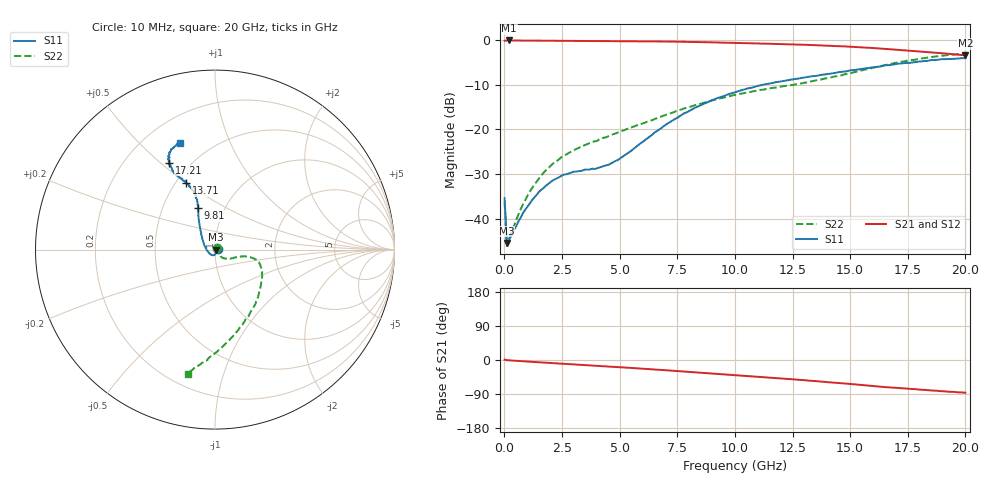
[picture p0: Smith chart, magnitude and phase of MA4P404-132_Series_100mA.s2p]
! AWR Design Environment (9226) Thu Aug 19 02:30:18 2021
! Document = '100mA'
! nPorts: 2, nXvals: 201
# GHz S DB R 50
!Freq DBS11 AngS11 DBS21 AngS21 DBS12 AngS12 DBS22 AngS22
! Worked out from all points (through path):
!   201 points, 10 MHz to 20 GHz, reference 50 ohm
!   highest |S21| = -0.10 dB at 210 MHz (marker M1); lowest = -3.4 dB at 20 GHz (marker M2)
!   group delay of S21, straight-line fit = 12.2 ps
!   lowest |S11| = -45.5 dB at 110 MHz (marker M3), VSWR 1.01, Z = 50.5 - j0.0632 ohm
!   |S11| at or under -10 dB: start of sweep to 11.23 GHz
!   |S22| runs from -46.2 to -3.0 dB; largest |S21 - S12| = 0.034
!   S11 on the Smith chart (normalised r, x): 10 MHz: 1.03, +0.01; 9.81 GHz: 0.75, +0.37; 13.71 GHz: 0.56, +0.50; 17.21 GHz: 0.39, +0.54; 20 GHz: 0.34, +0.67
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0.01  -35.40 19.9  -0.17 1.0  -0.15 0.7  -36.31 48.5
0.11  -45.45 -6.7  -0.10 -0.5  -0.09 -0.5  -46.16 -8.1
0.21  -44.72 -16.0  -0.10 -0.9  -0.09 -0.9  -44.45 -12.8
0.81  -38.73 -52.3  -0.12 -3.4  -0.11 -3.3  -36.76 -39.9
1.11  -36.56 -63.1  -0.14 -4.6  -0.12 -4.4  -33.86 -44.8
1.61  -33.52 -75.7  -0.16 -6.4  -0.15 -6.2  -30.27 -47.6
2.51  -30.30 -97.2  -0.20 -9.7  -0.18 -9.3  -26.10 -50.1
3.41  -29.16 -120.8  -0.22 -13.0  -0.20 -12.5  -23.72 -46.0
4.01  -28.76 -139.4  -0.22 -15.3  -0.21 -14.7  -22.63 -41.9
4.91  -26.90 -176.1  -0.24 -18.6  -0.24 -17.9  -20.74 -33.6
6.71  -20.08 136.7  -0.31 -25.8  -0.30 -25.0  -17.34 -17.5
7.81  -16.37 123.7  -0.40 -30.5  -0.40 -29.4  -15.30 -12.7
9.81  -12.00 112.5  -0.61 -38.9  -0.60 -37.5  -12.51 -13.9
10.01  -11.69 111.1  -0.63 -39.9  -0.62 -38.3  -12.30 -14.1
11.71  -9.52 110.1  -0.87 -47.3  -0.81 -45.6  -10.69 -26.1
13.41  -8.09 112.9  -1.14 -55.2  -1.05 -53.5  -9.15 -45.6
13.71  -7.84 113.3  -1.20 -56.9  -1.11 -55.0  -8.87 -49.5
14.81  -7.03 116.1  -1.44 -62.2  -1.33 -60.5  -7.63 -63.4
16.71  -5.62 118.1  -2.06 -72.4  -1.94 -70.7  -5.41 -84.8
17.21  -5.24 117.6  -2.25 -74.6  -2.15 -73.3  -4.89 -88.9
18.71  -4.45 115.1  -2.87 -81.0  -2.85 -80.5  -3.68 -98.3
20  -4.06 108.2  -3.41 -86.5  -3.51 -85.6  -3.01 -102.3
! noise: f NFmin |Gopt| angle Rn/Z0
0.01  0  1  0  2e-20
2.21  0  1  0  2e-20
4.41  0  1  0  2e-20
6.61  0  1  0  2e-20
8.81  0  1  0  2e-20
11.11  0  1  0  2e-20
13.31  0  1  0  2e-20
15.51  0  1  0  2e-20
17.71  0  1  0  2e-20
20  0  1  0  2e-20
